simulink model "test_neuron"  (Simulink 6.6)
settings: Solver=ode45  StartTime=0.0  StopTime=5e-6  RelTol=1e-3
libraries: simulink x1

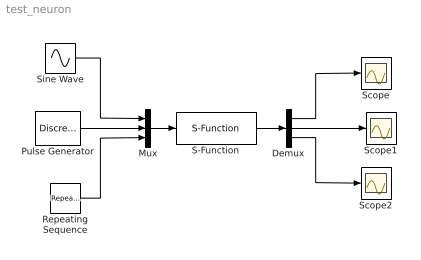
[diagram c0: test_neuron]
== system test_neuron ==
  Demux : Demux  Outputs=3
  Mux : Mux  Inputs=3
  Pulse Generator : DiscretePulseGenerator  PulseType=Time based  Amplitude=2  Period=.5e-6  PulseWidth=50
  Repeating Sequence : simulink/Sources/Repeating Sequence  SystemSampleTime=-1  rep_seq_t=[0 2e-6]  rep_seq_y=[0 3]
  S-Function : S-Function  FunctionName=neuron_node_s  Parameters=1e-8 3 'param.dat' 'in_b.dat'
  Scope : Scope
  Scope1 : Scope
  Scope2 : Scope
  Sine Wave : Sin  Amplitude=5  Frequency=2*pi*1e6  SampleTime=0
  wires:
  Mux/1 -> S-Function/1
  S-Function/1 -> Demux/1
  Pulse Generator/1 -> Mux/2
  Sine Wave/1 -> Mux/1
  Repeating Sequence/1 -> Mux/3
  Demux/1 -> Scope/1
  Demux/2 -> Scope1/1
  Demux/3 -> Scope2/1
